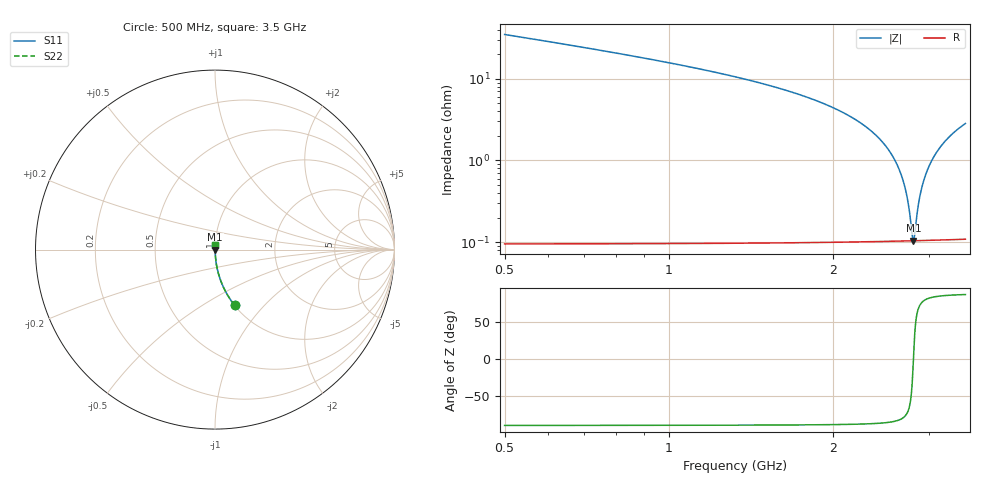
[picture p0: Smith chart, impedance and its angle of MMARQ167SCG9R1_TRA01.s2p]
! MMARQ167SCG9R1_TRA01  S-PARAMETER MODEL  ( General Type )
! Model Generated by TAIYO YUDEN Corporation (http://www.ty-top.com)
! Version 1.0
! TAIYO YUDEN Control No. 180601
! Copyright(c) 2018 TAIYO YUDEN CO.,LTD. All Rights Reserved.
! Product Description (link to TY-COMPAS)
! https://ds.yuden.co.jp/TYCOMPAS/or/detail?pn=MMARQ167SCG9R1CTRA01&u=M
! Products Name : Multilayer Ceramic Capacitors
! Characteristics :
!  Capacitance : 9.1 pF , Rated Voltage : 250V , TCC : CG / C0G
!  Case Size : 1.6 x 0.8 / 0.063 x 0.031 [mm/inch] , Thickness : 0.7 / 0.028 [mm/inch]
!  (Conditions: Temperature = 25 degC , DC Bias Current/Voltage = 0A / 0V)
! External Node Assignments :
!  1  o---| |---o  2
! GND o---------o GND
! Frequency Range : 500MHz  -  3500MHz  [ 401 STEP ]
# MHz S RI R 50
! Freq[MHz].  S11 Real  S11 Imag  S21 Real  S21 Imag  S12 Real  S12 Imag  S22 Real  S22 Imag
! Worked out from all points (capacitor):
!   401 points, 500 MHz to 3.5 GHz, reference 50 ohm
!   read as one part in series: C = 8.84 pF near 515 MHz
!   lowest |Z| = 104 mohm at 2.81 GHz (marker M1)
!   series resonance near 2.81 GHz, so ESL is about 360 pH
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500  0.109 -0.3103  0.891 0.3103  0.891 0.3103  0.109 -0.3103
725  0.0518 -0.2195  0.9482 0.2195  0.9482 0.2195  0.0518 -0.2195
1002.5  0.0248 -0.1526  0.9752 0.1526  0.9752 0.1526  0.0248 -0.1526
1505  0.00817 -0.0845  0.9918 0.0845  0.9918 0.0845  0.00817 -0.0845
2000  0.00296 -0.0442  0.997 0.0442  0.997 0.0442  0.00296 -0.0442
2292.5  0.0017 -0.0262  0.9983 0.0262  0.9983 0.0262  0.0017 -0.0262
2502.5  0.00124 -0.0148  0.9988 0.0148  0.9988 0.0148  0.00124 -0.0148
2607.5  0.00112 -0.00957  0.9989 0.00957  0.9989 0.00957  0.00112 -0.00957
2690  0.00106 -0.00558  0.9989 0.00558  0.9989 0.00558  0.00106 -0.00558
2742.5  0.00105 -0.00311  0.999 0.00311  0.999 0.00311  0.00105 -0.00311
2765  0.00104 -0.00207  0.999 0.00207  0.999 0.00207  0.00104 -0.00207
2795  0.00104 -0.000689  0.999 0.000689  0.999 0.000689  0.00104 -0.000689
2810  0.00104 -5.46e-06  0.999 5.46e-06  0.999 5.46e-06  0.00104 -5.46e-06
2825  0.00104 0.000675  0.999 -0.000675  0.999 -0.000675  0.00104 0.000675
2862.5  0.00105 0.00236  0.999 -0.00236  0.999 -0.00236  0.00105 0.00236
2900  0.00106 0.00402  0.9989 -0.00402  0.9989 -0.00402  0.00106 0.00402
2945  0.00108 0.00599  0.9989 -0.00599  0.9989 -0.00599  0.00108 0.00599
3005  0.00113 0.00857  0.9989 -0.00857  0.9989 -0.00857  0.00113 0.00857
3095  0.00121 0.0124  0.9988 -0.0124  0.9988 -0.0124  0.00121 0.0124
3200  0.00134 0.0166  0.9987 -0.0166  0.9987 -0.0166  0.00134 0.0166
3342.5  0.00157 0.0223  0.9984 -0.0223  0.9984 -0.0223  0.00157 0.0223
3500  0.00189 0.0282  0.9981 -0.0282  0.9981 -0.0282  0.00189 0.0282
